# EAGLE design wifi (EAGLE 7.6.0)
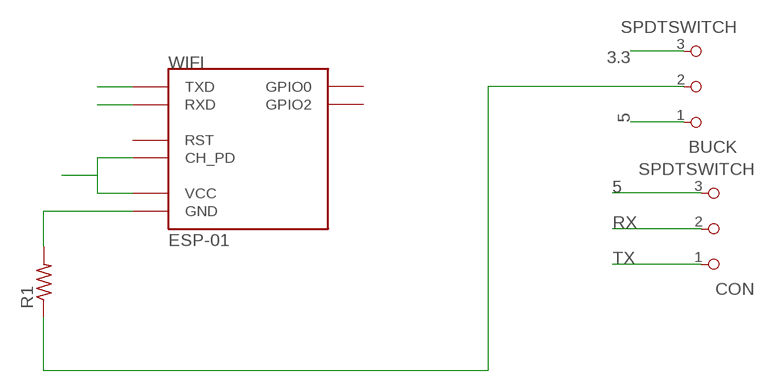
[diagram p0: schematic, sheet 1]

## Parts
BUCK  SPDTSWITCH  [SPDTSWITCH]
CON  SPDTSWITCH  [SPDTSWITCH]
R1  RES-US1206FAB  [R1206FAB]
WIFI  ESP-01  [ESP-01]

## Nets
3.3: BUCK.3 WIFI.CH_PD WIFI.VCC
5: BUCK.1 CON.3
N$1: BUCK.2 R1.1
N$2: R1.2 WIFI.GND
RX: CON.2 WIFI.RX(RXD)
TX: CON.1 WIFI.TX(TXD)
Unconnected: WIFI.GPIO0 WIFI.GPIO2 WIFI.RST

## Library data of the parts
BUCK CON = fab:SPDTSWITCH
R1 = fab:RES-US: Resistor (US Symbol)
WIFI = esp8266modules:ESP-01: ESP8266 Wifi Module ESP-01; DIMENSIONS: 14.3 x 24.8 mm; PINS: 8; PITCH: 0.1" / 2.54 mm

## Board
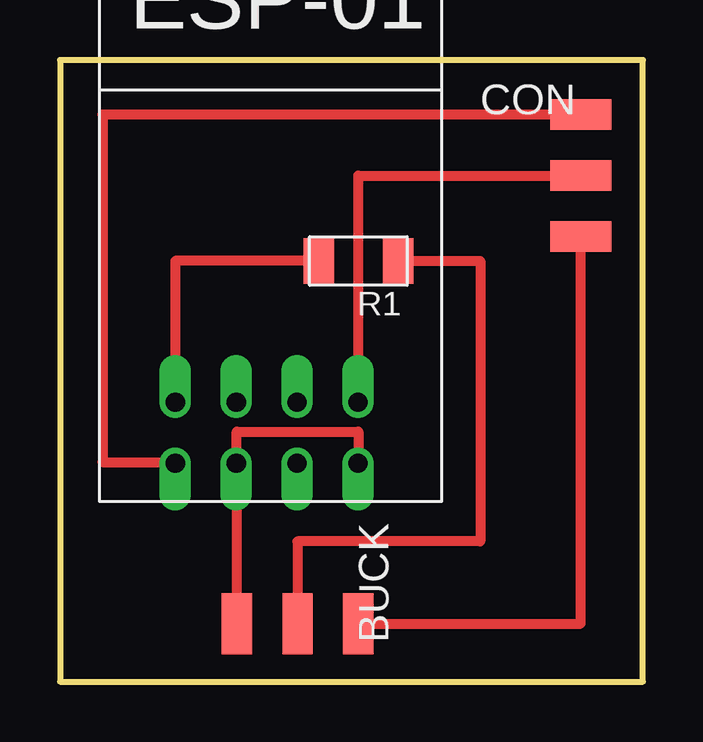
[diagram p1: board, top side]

Size 24.31 x 25.9 mm. Coordinates in mm from the lower left corner, seen from the top.
Outline: 0,0 24.31,0 24.31,25.9 0,25.9 0,0
Copper layers (1*16): Top 0.035mm / dielectric 1.5mm / Bottom 0.035mm
Design rules "default *": minimum track width 16mil, minimum drill 24mil, track to track 16mil, track to pad 16mil, pad to pad 8mil, via to via 8mil, smd to smd 8mil, copper to edge 40mil, drill to drill 8mil, minimum pad ring 10mil, minimum via ring 8mil, stop-mask expansion 4mil, vias tented up to drill 0mil, thermal gap 10mil

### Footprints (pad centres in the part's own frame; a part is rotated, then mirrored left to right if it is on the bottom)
SPDTSWITCH = smd 2.54 x 1.27: 1 0.38,2.54; 2 0.38,0; 3 0.38,-2.54
R1206FAB = smd 1.27 x 1.905: 1 -1.651,0; 2 1.651,0
ESP-01 = drill 0.8 offset: CH_PD -1.285,-8.178; GND -3.825,-5.638; GPIO0 1.255,-5.638; GPIO2 -1.285,-5.638; RST 1.255,-8.178; RX 3.795,-5.638; TX -3.825,-8.178; VCC 3.795,-8.178

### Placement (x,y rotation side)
BUCK  9.91,2.79 270 top
CON  21.34,21.08 0 top
R1  12.45,17.53 180 top
WIFI  8.64,17.27 0 top

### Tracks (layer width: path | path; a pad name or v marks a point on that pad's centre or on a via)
3.3
  Top 0.406: WIFI.CH_PD 7.37,9.1 | 7.37,9.1 BUCK.3 | 7.37,9.1 7.37,10.41 12.45,10.41 12.45,9.1 WIFI.VCC
5
  Top 0.406: BUCK.1 21.72,2.41 CON.3
N$1
  Top 0.406: R1.1 17.53,17.53 17.53,5.84 9.91,5.84 BUCK.2
N$2
  Top 0.406: R1.2 4.81,17.53 WIFI.GND
RX
  Top 0.406: CON.2 12.45,21.08 12.45,11.63 WIFI.RX
TX
  Top 0.406: CON.1 1.78,23.62 1.78,9.14 4.81,9.14 WIFI.TX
